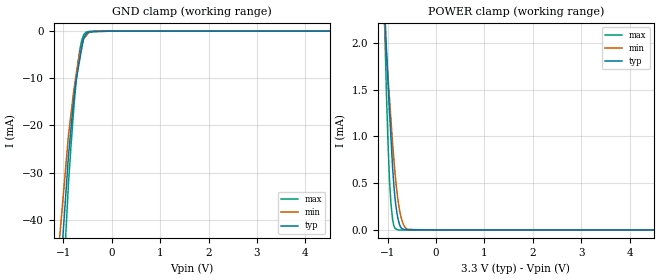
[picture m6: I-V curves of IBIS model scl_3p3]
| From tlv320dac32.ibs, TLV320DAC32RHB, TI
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|   scl_3p3 Model
[Model]   scl_3p3
Model_type   Input
Vinl = 0.99
Vinh = 2.31
|   typ   min   max
|   (nom PVT)   (fast PVT)   (slow PVT)
|C_comp from frequency sweep method (F=0.4MHz)
|Average
|C_comp   3.566e-12   3.518e-12   3.605e-12
|C_comp from LC tank measurement(L=1nH)
|Average
|Resonant Frequency(Hz)   4.780e+09   4.790e+09   4.770e+09
C_comp   1.110e-12   1.105e-12   1.114e-12
[model spec]
|subparameter   typ   min   max
Vinl   0.99   0.90   1.08
Vinh   2.31   2.10   2.52
| Where nom  PVT is Nominal Process, 3.3V, 45C
|   Fast PVT is Strong Process,  3.6V, -40C
|   Slow PVT is Weak Process,   3V, 105C
[Voltage Range]   3.3   3   3.6
|Ambient Temperature   25   85   -40
|Junction Temperature
[Temperature Range]   45   105   -40
[Power Clamp Reference]   3.3   3   3.6
[GND Clamp Reference]   0   0   0
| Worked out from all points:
|   GND clamp passes 1 mA (typ) near -0.56 V on its own axis
|   POWER clamp passes 1 mA (typ) near -0.93 V on its own axis
[GND Clamp]
|   Voltage   I(typ)   I(min)   I(max)
-3.3V     -1.46A     -1.307A    -1.662A
-1.49V    -115mA     -92.71mA   -147.7mA
-897.6mV  -26.39mA   -22.11mA   -32.41mA
-792mV    -15.05mA   -13.04mA   -16.99mA
-745.8mV  -10.84mA   -9.703mA   -11.43mA
-702mV    -8.268mA   -6.817mA   -7.045mA
-622.8mV  -3.616mA   -3.166mA   -1.957mA
-590.7mV  -1.731mA   -1.919mA   -1.015mA
-532.8mV  -615uA     -1.015mA   -208.3uA
-465mV    -195.4uA   -194.6uA   -64.22uA
-285mV    -119.2uA   -2.502uA   -4.665uA
6.6V      0A         0A         0A
[POWER Clamp]
|   Voltage   I(typ)   I(min)   I(max)
-3.3V     32.08mA    22.4mA     56.05mA
-1.089V   2.679mA    2.39mA     2.744mA
-1.03V    1.983mA    1.906mA    1.532mA
-993.6mV  1.586mA    1.634mA    934uA
-964.8mV  1.288mA    1.419mA    561.5uA
-932.4mV  983.8uA    1.176mA    280.4uA
-896.4mV  648.9uA    907.5uA    104uA
-864.6mV  429.3uA    705.3uA    36.05uA
-792mV    130.4uA    335uA      1.308uA
-681mV    8.006uA    64.67uA    29.88nA
-585mV    3.401uA    6.441uA    18.04nA
6.6V      0A         0A         0A
